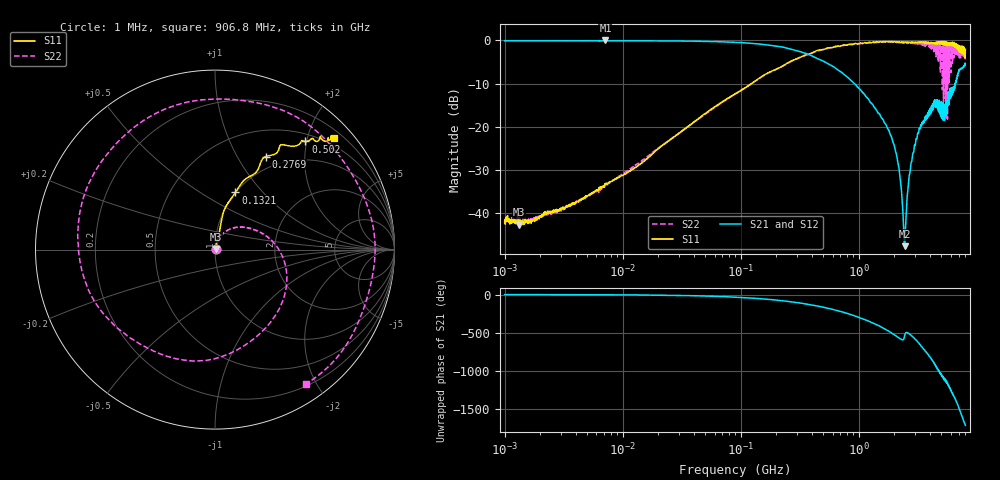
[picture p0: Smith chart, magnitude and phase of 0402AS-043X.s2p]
!s-Parameter Generated by FASTRON Sdn. Bhd.
!FASTRON P/N : 0402AS-043X
!Keysight Technologies: E5071C_MY46733604_B.14.02
!Date: Mon Dec 01 10:46:51 2025
!Version  :Rev00  Mon Dec 01 10:46:51 2025
!Data & Calibration Information:
!Freq  S11:SOLT2(ON)  S21:SOLT2(ON)  S12:SOLT2(ON)  S22:SOLT2(ON)
!PortZ  Port1:50+j0  Port2:50+j0
!When reading reference impedance value at option line is always used.
! Remarks : This data is being provided solely for informational purposes.
# Hz S dB R 50
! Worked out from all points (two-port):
!   1601 points, 1 MHz to 8 GHz, reference 50 ohm
!   highest |S21| = 0.00 dB at 7.138 MHz (marker M1); lowest = -47.6 dB at 2.443 GHz (marker M2)
!   |S21| within 3 dB of the highest: start of sweep to 355.6 MHz
!   lowest |S11| = -42.6 dB at 1.323 MHz (marker M3), VSWR 1.01, Z = 50.6 + j0.406 ohm
!   |S11| at or under -10 dB: start of sweep to 123.2 MHz
!   |S22| runs from -42.6 to -0.1 dB; largest |S21 - S12| = 0.013
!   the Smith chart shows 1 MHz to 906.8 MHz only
!   S11 on the Smith chart (normalised r, x): 1 MHz: 1.01, +0.01; 132.1 MHz: 1.00, +0.72; 276.9 MHz: 0.83, +1.32; 502 MHz: 0.63, +1.98; 906.8 MHz: 0.35, +2.49
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1000000  -42.00 25.6  -0.07 -0.4  -0.07 -0.4  -41.30 24.7
1323440  -42.60 32.7  -0.07 -0.5  -0.07 -0.5  -41.70 19.3
4479405  -36.80 58.6  -0.08 -1.9  -0.07 -1.8  -36.80 59.4
7138274  -33.10 64.8  0.00 -3.0  -0.05 -2.7  -33.20 63.7
2.00676e7  -25.00 75.6  -0.10 -7.9  -0.10 -7.8  -24.90 70.3
8.994653e7  -12.30 76.2  -0.42 -34.1  -0.41 -34.1  -12.40 28.2
1.320665e8  -9.42 70.3  -0.72 -49.4  -0.72 -49.4  -9.43 4.7
2.7692e8  -4.59 61.4  -2.13 -98.7  -2.12 -98.6  -4.64 -82.5
4.006501e8  -2.93 53.9  -3.56 -138.0  -3.54 -138.0  -2.84 -152.0
5.019708e8  -2.10 50.1  -4.80 -167.0  -4.79 -167.0  -2.03 155.0
9.068124e8  -0.84 43.1  -9.80 84.8  -9.80 84.7  -0.87 -56.1
1.13703e9  -0.49 46.7  -12.80 28.5  -12.80 28.4  -0.66 -173.0
1.334081e9  -0.36 51.4  -15.20 -16.6  -15.20 -16.6  -0.52 90.8
1.542898e9  -0.31 57.5  -17.70 -62.8  -17.70 -62.9  -0.35 -8.3
1.7949e9  -0.24 64.0  -20.80 -120.0  -20.80 -120.0  -0.40 -130.0
2.082516e9  -0.32 70.9  -26.30 175.0  -26.30 175.0  -0.48 88.0
2.44288e9  -0.54 77.0  -47.60 177.0  -47.60 179.0  -0.37 -85.4
2.824359e9  -0.52 87.7  -27.60 176.0  -27.60 176.0  -0.33 93.3
3.183204e9  -0.38 97.5  -21.50 92.0  -21.50 91.7  -0.58 -91.0
3.548043e9  -0.40 109.0  -18.60 3.5  -18.60 3.2  -1.18 81.4
3.933151e9  -0.67 114.0  -16.20 -81.5  -16.20 -82.0  -1.50 -92.4
8e9  -2.00 -113.0  -5.38 86.4  -5.40 86.0  -4.41 122.0
